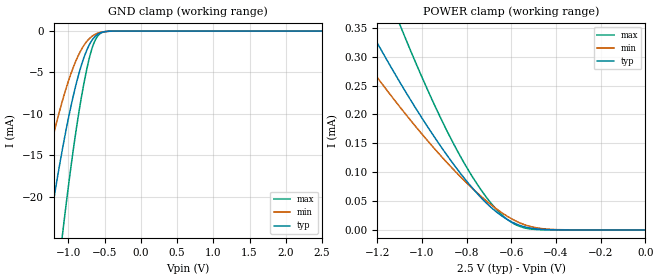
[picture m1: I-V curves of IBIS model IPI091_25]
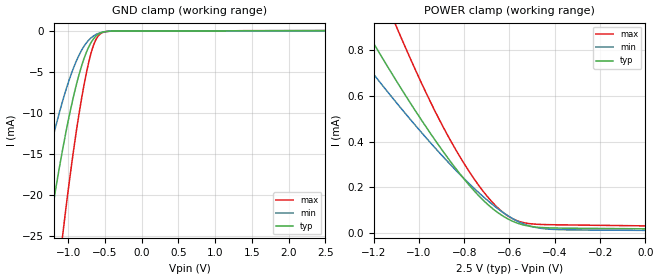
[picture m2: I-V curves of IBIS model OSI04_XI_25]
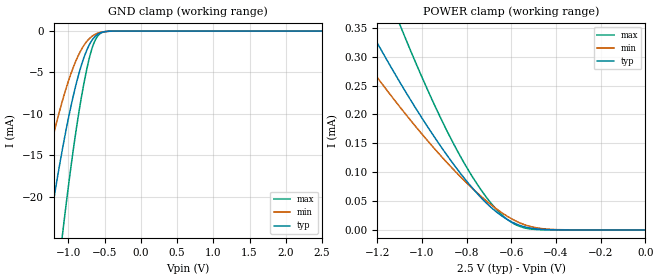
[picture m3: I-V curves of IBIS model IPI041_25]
| TEXAS INSTRUMENTS INCORPORATED
| Connectivity Solutions Group
| IBIS Model of TL16C2550RHB_25V
| 2550RHB_25V
| This file contains package information for the following:
|  RHB 32-pin (QFN) package as [Component] 2550RHB_25V
| This device can be powered at the following Vccs:
|  2.5 volt Vcc
| This file provides unique models under the [Model Selector] for each Vcc.
| For operation at a specific Vcc, select the appropriate model after each
| [Model Selector] keyword.
[IBIS Ver]   3.2
[Comment char]  |_char
[File Name]   2550RHB_25v.ibs
[File Rev]   1 | a
[Date]   August 7, 2006
[Source]   Data created from TI-SPICE simulations at TI-CONN.
[Notes]   The following is an IBIS list for the 2550RHB_25V.
   Please contact s-ly@ti.com with questions and
   comments concerning CONN IBIS models.
[Disclaimer] Property of Texas Instruments Incorporated.  Unauthorized
   reproduction and/or distribution is strictly prohibited.
   This product is protected under copyright law.
   Created  2003, (C) Copyright  2003, Texas Instruments
   Incorporated, All Rights Reserved
   UNLESS THERE IS A SIGNED, WRITTEN AGREEMENT TO THE
   CONTRARY, TEXAS INSTRUMENTS (TI) IS PROVIDING THE IBIS
   MODELS  AND WITHOUT ANY WARRANTY, EXPRESSED OR
   IMPLIED.  TI assumes no liability for:
   1) the accuracy of the IBIS models provided to your
   company;
   2) the proper functioning of these IBIS Models in your
   design or for any resulting applications; or
   3) infringement of patents, copyrights or intellectual
   property rights resulting from your use of these IBIS
   models.
   TI provides IBIS Models as a service to our customers.
   You and your company shall not distribute, sell or give
   these models to anyone else without prior written
   permission from TI.
   TI reserves the right to make changes to our products or
   to discontinue any semiconductor product or service
   without notice, and advises our customers to obtain the
   latest version of relevant information to verify, before
   placing orders, that the information being relied on is
   current.
   Please be aware that your receipt and use of the IBIS
   information provided shall serve as acceptance of these
   terms and conditions.  If you do not accept these terms,
   you should return or destroy the IBIS models and any
   other accompanying information immediately.
| Component 2550_25V_QFN 32-pin RHB
[Component]   2550RHB_25V
[Manufacturer]   Texas Instruments, Inc.
[Package]
|   typ   min   max
R_pkg   0.12388   0.10657   0.14120
L_pkg   1.56476n   1.31872n   1.81080n
C_pkg   0.11271p   0.09406p   0.13136p
[Pin]   signal_name   model_name   R_pin   L_pin   C_pin
1   D6   IPI04_OPJ43   0.14120   1.81080n   0.13136p
2   D7   IPI04_OPJ43   0.12425   1.57381n   0.11746p
3   RXB   IPI041   0.11263   1.41203n   0.10400p
4   RXA   IPI041   0.10692   1.33284n   0.09561p
5   TXA   OPJ430   0.10719   1.33655n   0.09556p
6   TXB   OPJ430   0.11347   1.42368n   0.10187p
7   CSA   IPI041   0.12187   1.54058n   0.11146p
8   CSB   IPI041   0.13812   1.76758n   0.12177p
9   NC   NC
10   XTAL1   OSI04_XI   0.11688   1.46877n   0.10136p
11   XTAL2   OSI04   0.10853   1.35128n   0.09807p
12   IOW   IPI041   0.10671   1.32444n   0.09406p
13   GND   GND   0.10950   1.36218n   0.09511p
14   IOR   IPI041   0.11586   1.44976n   0.09980p
15   RTSB   OPJ430   0.12065   1.51617n   0.10792p
16   CTSB   IPI041   0.13618   1.73254n   0.11898p
17   NC   NC
18   A2   IPI041   0.11794   1.47628n   0.10220p
19   A1   IPI041   0.10905   1.35202n   0.09922p
20   A0   IPI041   0.10667   1.31872n   0.09658p
21   INTB   OPJ430   0.11105   1.37994n   0.10092p
22   INTA   OPJ430   0.12147   1.52573n   0.10799p
23   RTSA   OPJ430   0.12769   1.61294n   0.11024p
24   RESET   IPI091   0.13662   1.73818n   0.11596p
25   CTSA   IPI041   0.13407   1.70317n   0.11232p
26   VCC   POWER   0.13028   1.65014n   0.11280p
27   D0   IPI04_OPJ43   0.12020   1.51001n   0.10862p
28   D1   IPI04_OPJ43   0.11017   1.37138n   0.10102p
29   D2   IPI04_OPJ43   0.10657   1.32284n   0.09730p
30   D3   IPI04_OPJ43   0.11011   1.37349n   0.10094p
31   D4   IPI04_OPJ43   0.12009   1.51391n   0.10606p
32   D5   IPI04_OPJ43   0.14072   1.80276n   0.12325p
| Model IPI091
[Model Selector]   IPI091
IPI091_25   2.5 volt Vcc
| Model OSI04_XI
[Model Selector]   OSI04_XI
OSI04_XI_25   2.5 volt Vcc
| Model IPI041
[Model Selector]   IPI041
IPI041_25   2.5 volt Vcc
| Model IPI04_OPJ43
[Model Selector]   IPI04_OPJ43
IPI04_OPJ43_25   2.5 volt Vcc
| Model OPJ430
[Model Selector]   OPJ430
OPJ430_25   2.5 volt Vcc
| Model OSI04
[Model Selector]   OSI04
OSI04_25   2.5 volt Vcc
| Models and submodels in the file (6): IPI091_25 (Input), OSI04_XI_25 (Input), IPI041_25 (Input), IPI04_OPJ43_25 (I/O), OPJ430_25 (3-state), OSI04_25 (3-state)
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[Model]   IPI091_25
Model_type  Input
Vinl = 0
Vinh = 2.5
| variable   typ   min   max
C_comp   1.09pF   0.97pF   1.21pF
[Temperature Range]   40   125   -40
| Ambient temperature   25   110   -40
[Voltage range]   2.5   2.3   2.7
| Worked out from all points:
|   GND clamp passes 1 mA (typ) near -0.66 V on its own axis
|   POWER clamp passes 1 mA (typ) near -2.03 V on its own axis
[GND Clamp]
| IPI091_25
|   Voltage   I(typ)   I(min)   I(max)
-2.5V     -115mA     -79.72mA   -164.4mA
-1.485V   -37.43mA   -23.94mA   -59.12mA
-1.265V   -23.92mA   -14.77mA   -39.38mA
-1.08V    -14.2mA    -8.377mA   -24.56mA
-1.065V   -13.5mA    -7.923mA   -23.45mA
-955mV    -8.737mA   -4.937mA   -15.83mA
-830mV    -4.417mA   -2.392mA   -8.532mA
-730mV    -2.005mA   -1.091mA   -3.99mA
-635mV    -690.9uA   -415.3uA   -1.203mA
-560mV    -221.4uA   -161.8uA   -300.1uA
-440mV    -21.14uA   -26.42uA   -19.38uA
2.5V      179.9pA    7.156nA    49.54pA
[POWER Clamp]
| IPI091_25
|   Voltage   I(typ)   I(min)   I(max)
-2.5V     1.454mA    1.097mA    2.083mA
-1.36V    439.4uA    350.2uA    624.8uA
-1.235V   348.4uA    282.4uA    491.3uA
-1.095V   253.5uA    211.2uA    352uA
-1.075V   240.6uA    201.5uA    333.1uA
-945mV    161.4uA    141.3uA    217.5uA
-830mV    99.28uA    93.13uA    129uA
-720mV    49.87uA    53.05uA    61.07uA
-630mV    21.07uA    26.64uA    21.99uA
-550mV    6.466uA    10.43uA    4.583uA
-465mV    1.046uA    2.442uA    370.2nA
-31.11fV  179.9pA    1.684nA    54.24pA
[Model]   OSI04_XI_25
Model_type  Input
Vinl = 0
Vinh = 2.5
| variable   typ   min   max
C_comp   1.81pF   1.12pF   2.40pF
[Temperature Range]   40   125   -40
| Ambient temperature   25   110   -40
[Voltage range]   2.5   2.3   2.7
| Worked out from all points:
|   GND clamp passes 1 mA (typ) near -0.66 V on its own axis
|   POWER clamp passes 1 mA (typ) near -1.30 V on its own axis
[GND Clamp]
| OSI04_XI_25
|   Voltage   I(typ)   I(min)   I(max)
-2.5V     -117.2mA   -81mA      -167.9mA
-1.48V    -38.04mA   -24.27mA   -60.11mA
-1.26V    -24.32mA   -15mA      -40.01mA
-1.075V   -14.44mA   -8.535mA   -24.92mA
-1.06V    -13.72mA   -8.076mA   -23.8mA
-930mV    -8.097mA   -4.582mA   -14.76mA
-815mV    -4.206mA   -2.33mA    -8.111mA
-710mV    -1.776mA   -1.037mA   -3.434mA
-625mV    -669.3uA   -465.2uA   -1.116mA
-545mV    -205.3uA   -194.2uA   -270.4uA
-430mV    -40.49uA   -47uA      -53.13uA
2.5V      19.05uA    13.35uA    29.56uA
[POWER Clamp]
| OSI04_XI_25
|   Voltage   I(typ)   I(min)   I(max)
-2.5V     3.431mA    2.617mA    4.916mA
-1.355V   1.099mA    896.3uA    1.535mA
-1.24V    898.6uA    746.4uA    1.242mA
-1.22V    864.6uA    720.9uA    1.193mA
-1.095V   659.2uA    565.9uA    893.7uA
-935mV    416.4uA    380.2uA    546.2uA
-830mV    273.7uA    268.3uA    352.9uA
-720mV    148uA      163.2uA    188uA
-625mV    72.54uA    88.13uA    88.07uA
-555mV    40.52uA    47.83uA    50.59uA
-465mV    25.13uA    21.75uA    38.3uA
-31.11fV  19.05uA    12.27uA    31.94uA
[Model]   IPI041_25
Model_type  Input
Vinl = 0
Vinh = 2.5
| variable   typ   min   max
C_comp   1.10pF   0.98pF   1.21pF
[Temperature Range]   40   125   -40
| Ambient temperature   25   110   -40
[Voltage range]   2.5   2.3   2.7
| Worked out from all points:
|   GND clamp passes 1 mA (typ) near -0.66 V on its own axis
|   POWER clamp passes 1 mA (typ) near -2.03 V on its own axis
[GND Clamp]
| IPI041_25
|   Voltage   I(typ)   I(min)   I(max)
-2.5V     -115mA     -79.72mA   -164.4mA
-1.485V   -37.43mA   -23.94mA   -59.12mA
-1.265V   -23.92mA   -14.77mA   -39.38mA
-1.08V    -14.2mA    -8.377mA   -24.56mA
-1.065V   -13.5mA    -7.923mA   -23.45mA
-955mV    -8.737mA   -4.937mA   -15.83mA
-830mV    -4.417mA   -2.392mA   -8.532mA
-730mV    -2.005mA   -1.091mA   -3.99mA
-635mV    -690.9uA   -415.3uA   -1.203mA
-560mV    -221.4uA   -161.8uA   -300.1uA
-440mV    -21.14uA   -26.42uA   -19.38uA
2.5V      179.9pA    7.156nA    49.54pA
[POWER Clamp]
| IPI041_25
|   Voltage   I(typ)   I(min)   I(max)
-2.5V     1.454mA    1.097mA    2.083mA
-1.36V    439.4uA    350.2uA    624.8uA
-1.235V   348.4uA    282.4uA    491.3uA
-1.095V   253.5uA    211.2uA    352uA
-1.075V   240.6uA    201.5uA    333.1uA
-945mV    161.4uA    141.3uA    217.5uA
-830mV    99.28uA    93.13uA    129uA
-720mV    49.87uA    53.05uA    61.07uA
-630mV    21.07uA    26.64uA    21.99uA
-550mV    6.466uA    10.43uA    4.583uA
-465mV    1.046uA    2.442uA    370.2nA
-31.11fV  179.9pA    1.684nA    54.24pA
